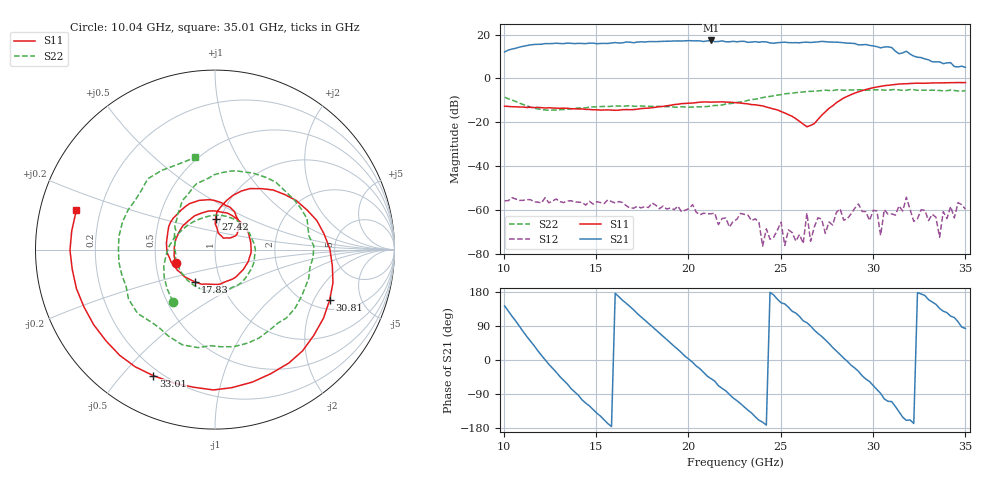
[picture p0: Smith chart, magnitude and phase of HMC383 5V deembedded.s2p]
!Hittite Microwave Corporation
!20 Alpha Road
!Chelmsford, MA 01824
!Tel: 978-250-3343
!Fax: 978-250-3373
!Device: HMC383, 12-30 GHz, Driver Amplifier Die
!Misc: Vcc = 5V, data includes two K connectors, Room
# MHZ S MA R 50
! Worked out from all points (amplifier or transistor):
!   126 points, 10.04 GHz to 35.01 GHz, reference 50 ohm
!   highest |S21| = 17.3 dB at 21.22 GHz (marker M1)
!   |S21| within 3 dB of that: 10.86 GHz to 30.27 GHz (19.41 GHz wide, 94.4 % of centre)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
!   unconditionally stable (mu >= 1): start of sweep to end of sweep
!   at 14.23 GHz: K = 49.12, MAG = 16.3 dB, |S12| = -56.6 dB
!   at 22.62 GHz: K = 101.05, MAG = 17.4 dB, |S12| = -64.3 dB
!   at 35.01 GHz: K = 69.10, MAG = 11.0 dB, |S12| = -59.7 dB
!   S11 on the Smith chart (normalised r, x): 10.04 GHz: 0.63, -0.10; 17.83 GHz: 0.76, -0.29; 27.42 GHz: 0.95, +0.34; 30.81 GHz: 2.44, -2.68; 33.01 GHz: 0.17, -0.61; 35.01 GHz: 0.11, +0.14
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10037.5  0.233 -160.6  4.032 142.7  0.00162 -18.5  0.373 -129.0
11036.25  0.223 143.8  5.411 75.5  0.001655 -24.4  0.255 175.1
12234.75  0.212 80.5  6.245 0.4  0.001908 -44.3  0.191 118.3
13433.25  0.209 27.3  6.41 -63.1  0.001596 -65.9  0.198 62.4
14232.25  0.202 -4.8  6.286 -105.0  0.001484 -76.6  0.213 25.4
16030  0.188 -68.0  6.593 176.2  0.001443 -96.0  0.236 -50.6
17827.75  0.211 -121.1  6.919 96.9  0.001134 -112.0  0.232 -113.6
18427  0.228 -138.8  6.975 71.0  0.001069 -114.1  0.23 -131.9
20025  0.273 172.3  7.307 1.9  0.00107 -143.5  0.22 -173.9
21223.5  0.288 136.4  7.363 -49.2  0.0008192 -145.6  0.236 164.0
22621.75  0.28 96.4  6.859 -107.2  0.0006114 -131.1  0.284 137.7
24219.75  0.223 58.6  6.805 -171.7  0.000371 161.6  0.382 105.4
25218.5  0.163 38.5  6.729 148.1  0.0001546 -17.0  0.445 79.2
26816.5  0.093 78.8  6.741 79.0  0.000405 -72.8  0.512 37.2
27415.75  0.173 88.8  6.918 53.2  0.0002932 -82.7  0.541 18.5
28214.75  0.317 71.9  6.64 14.4  0.001062 -77.4  0.548 -4.5
29013.75  0.464 45.7  6.268 -21.3  0.001095 -100.3  0.548 -28.5
30811.5  0.698 -23.9  5.273 -108.9  0.0008024 -116.4  0.536 -92.6
31011.25  0.715 -32.2  5.076 -109.7  0.0008139 -94.2  0.554 -99.7
31810.25  0.758 -65.7  4.181 -159.2  0.001955 -179.6  0.537 -130.9
33008.75  0.782 -116.0  2.663 159.2  0.0005728 109.8  0.538 179.7
35006.25  0.803 164.2  1.794 83.2  0.00104 72.7  0.525 102.1
